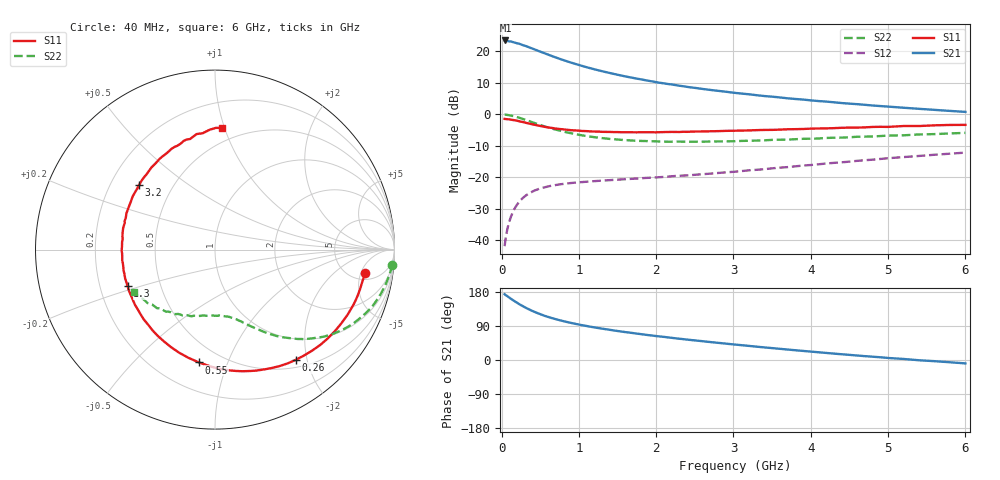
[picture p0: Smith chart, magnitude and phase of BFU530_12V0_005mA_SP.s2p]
! Filename:  P:\Prog\Test\Noise\ATS_data\Testdata_Net\03 Spar\BFU530_APG2013_40_A05_12p0V_005mA_SP_CM01_D.s2p
! Date/Time: Fri 26/Apr/2013 13:03:12
! BFU530_APG2013_40_A05_12p0V_1to25mA_SP_CM01_Bias4_R.s2p
! MDIF S-parameter v. bias file
! BFU530_APG2013_40_A05_12p0V_1to25mA_SP_CM01
! Date/time Wed Apr 24 20:41:12 2013
! VAR V_out= 12.0000
! VAR I_out= 5.0050
! VAR V_in= 0.8044
! VAR I_in= 0.0457
! Device data file deembeded for feedlines and parallel
! Original file: \03 Spar\BFU530_APG2013_40_A05_12p0V_005mA_SP_CM01_R.s2p
! Feed-files: PR047V01_250413_Feed1.s2p, PR047V01_250413_Feed2.s2p
! Parallel-file: PR047V01_250413_Par.s2p
# MHz S MA R 50
!  Freq-MHz  S11-mag  S11-arg  S21-mag  S21-arg  S12-mag  S12-arg  S22-mag  S22-arg
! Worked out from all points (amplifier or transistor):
!   98 points, 40 MHz to 6 GHz, reference 50 ohm
!   highest |S21| = 23.4 dB at 50 MHz (marker M1)
!   |S21| within 3 dB of that: start of sweep to 444.2 MHz
!   unconditionally stable (mu >= 1): 2.283 GHz to 4.413 GHz
!   at 300 MHz: K = 0.19, MSG = 23.9 dB, |S12| = -26.0 dB
!   at 1.6 GHz: K = 0.82, MSG = 16.3 dB, |S12| = -20.6 dB
!   at 6 GHz: K = 0.85, MSG = 6.5 dB, |S12| = -12.1 dB
!   S11 on the Smith chart (normalised r, x): 40 MHz: 6.55, -5.90; 260 MHz: 0.62, -1.81; 550 MHz: 0.38, -0.79; 1.3 GHz: 0.32, -0.18; 3.2 GHz: 0.32, +0.33; 6 GHz: 0.39, +0.98
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40  0.8453 -8.7  14.81 173.6  0.008118 82.6  0.9877 -4.9
50  0.8423 -10.9  14.82 171.4  0.0101 82.2  0.9878 -6.2
70  0.8377 -15.1  14.58 169.3  0.01402 80.4  0.9789 -8.9
140  0.8152 -30.2  14.06 159.0  0.02698 73.1  0.9443 -17.4
220  0.7804 -46.3  13.24 148.7  0.0397 65.3  0.8881 -26.1
260  0.7613 -53.8  12.72 143.8  0.04516 61.7  0.8579 -30.0
320  0.731 -64.6  12.03 137.1  0.05212 57.0  0.81 -35.3
400  0.6945 -77.4  11.01 129.3  0.05948 51.9  0.747 -41.1
550  0.6349 -98.2  9.354 117.1  0.06914 44.6  0.6458 -49.8
650  0.6079 -109.3  8.401 110.7  0.07396 41.4  0.5953 -54.2
750  0.5849 -119.2  7.585 105.1  0.07737 39.0  0.5518 -57.7
900  0.5595 -132.0  6.598 97.8  0.08143 36.5  0.5007 -62.2
1050  0.5438 -142.8  5.812 91.5  0.0844 34.9  0.4621 -66.0
1300  0.5275 -157.3  4.827 82.8  0.08882 33.8  0.4195 -71.0
1600  0.519 -171.8  3.992 73.7  0.09344 33.6  0.3898 -76.5
2050  0.5209 171.9  3.16 62.1  0.1008 34.9  0.3704 -84.3
2450  0.5307 158.8  2.667 52.7  0.1084 36.5  0.3669 -91.6
3100  0.551 141.6  2.134 39.2  0.1257 39.1  0.3782 -102.5
3200  0.5553 139.8  2.078 37.2  0.1294 39.4  0.3809 -103.9
4100  0.5962 119.3  1.621 20.4  0.1612 39.5  0.4134 -119.9
5200  0.6519 99.1  1.271 2.8  0.2099 35.2  0.4645 -138.7
6000  0.6796 86.5  1.092 -9.0  0.247 29.6  0.5081 -152.0
